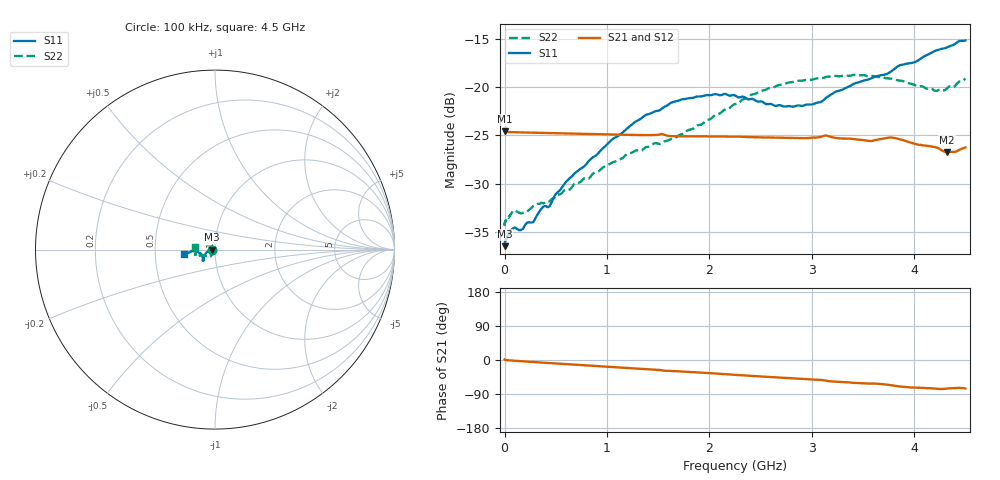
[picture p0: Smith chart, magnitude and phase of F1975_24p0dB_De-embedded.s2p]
! Integrated Device Technology
! Corporate Headquarters
! 6024 Silver Creek Valley Road
! San Jose, CA 95138  USA
! Phone:  1-408-284-8200
! Toll Free:  1-800-223-1366
! Webpage:  http://www.idt.com/
! Timing and RF Division
! 515 Groton Road, Suite 102
! Westford, MA 01886-6024
! Device:  F1975
! Description: 6-bit, 75 ohm, 0.5 dB Digital Step Attenuator
! Frequency:  5.0 MHz -  3.00 GHz
! Package:  4x4 mm QFN Plastic Package: 20 pin
! Ports:  2 RF, 11 DC
!  Pin  1  = D5 (16 dB)
!  Pin  2  = RF1  =  Port 1
!  Pin  3  = Serial Data In (DATA)
!  Pin  4  = Serial Clock (CLK)
!  Pin  5  = Serial Latch Enable (LE)
!  Pin  6  = VDD
!  Pin  7  = NC
!  Pin  8  = NC
!  Pin  9  = NC
!  Pin 10  = GND
!  Pin 11  = GND
!  Pin 12  = NC
!  Pin 13  = VMODE
!  Pin 14  = RF2  =  Port 2
!  Pin 15  = D4 (8 dB)
!  Pin 16  = D3 (4 dB)
!  Pin 17  = D2 (2 dB)
!  Pin 18  = NC
!  Pin 19  = D1 (1 dB)
!  Pin 20  = D0 (0.5 dB)
! State:  48
! Atten State:  24.0 dB
! Voltage:  +3.30 Volts
! Current:  0.595 mA
! Data:  The device was measured on a F1975 evaluation board which has
!  individual transmission lines to the RF pins.  Data was collected
!  using a calibrated network analyzer.  The evaluation board was
!  de-embedded using Automatic Fixture Removal (AFR).
!  The reference plane is the edge of the package pin.
! Misc:
!  Action Tracker AT0415
! Date Measured:  2018-02-08
! Date:  2018-03-26  MJV
! Note:
!  Integrated Device Technology supplies this data as a sample of measured
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# GHz S dB R 75
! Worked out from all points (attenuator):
!   291 points, 100 kHz to 4.5 GHz, reference 75 ohm
!   highest |S21| = -24.59 dB at 100 kHz (marker M1); lowest = -26.7 dB at 4.32 GHz (marker M2)
!   lowest |S11| = -36.5 dB at 100 kHz (marker M3), VSWR 1.03, Z = 72.8 + j0.00626 ohm
!   |S11| at or under -10 dB: start of sweep to end of sweep
!   |S22| runs from -34.4 to -18.7 dB; largest |S21 - S12| = 0.00015
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0.0001  -36.47 179.8  -24.59 1.2  -24.59 1.3  -34.38 -178.8
0.011  -35.78 -178.1  -24.65 -0.3  -24.65 -0.3  -33.81 -176.4
0.08  -34.64 -175.6  -24.67 -1.7  -24.67 -1.7  -32.84 -168.5
0.16  -34.79 -176.6  -24.70 -3.2  -24.70 -3.2  -33.09 -158.3
0.22  -34.02 -178.5  -24.71 -4.3  -24.71 -4.3  -32.89 -153.0
0.28  -33.98 -179.6  -24.73 -5.3  -24.73 -5.3  -32.32 -149.7
0.36  -32.58 -179.7  -24.75 -6.8  -24.75 -6.8  -31.98 -141.9
0.44  -32.33 -178.7  -24.77 -8.2  -24.77 -8.2  -31.84 -136.1
0.6  -29.81 -174.8  -24.81 -11.0  -24.81 -11.0  -30.60 -130.1
0.76  -28.36 -167.8  -24.85 -13.7  -24.84 -13.7  -29.60 -126.6
1.26  -23.73 -152.7  -24.96 -22.2  -24.96 -22.2  -26.69 -123.2
1.52  -22.37 -145.0  -24.89 -26.5  -24.89 -26.5  -25.89 -130.0
1.62  -21.66 -142.8  -25.09 -28.9  -25.08 -28.9  -25.41 -133.3
1.88  -20.98 -138.5  -25.11 -32.7  -25.11 -32.7  -23.97 -145.8
2.26  -20.93 -137.4  -25.13 -39.2  -25.13 -39.2  -21.75 -157.0
2.64  -21.95 -147.6  -25.24 -45.7  -25.23 -45.7  -19.98 -158.8
3.02  -21.74 -164.3  -25.23 -51.7  -25.23 -51.7  -19.20 -159.9
3.42  -19.63 -175.7  -25.41 -60.4  -25.41 -60.4  -18.74 -164.4
3.76  -18.50 -176.0  -25.23 -66.0  -25.23 -66.0  -19.13 -170.0
4.2  -16.28 -173.0  -26.22 -75.4  -26.21 -75.4  -20.39 178.5
4.32  -15.91 -172.5  -26.74 -75.4  -26.73 -75.4  -20.16 176.1
4.5  -15.19 -172.3  -26.26 -75.2  -26.25 -75.2  -19.11 173.6
